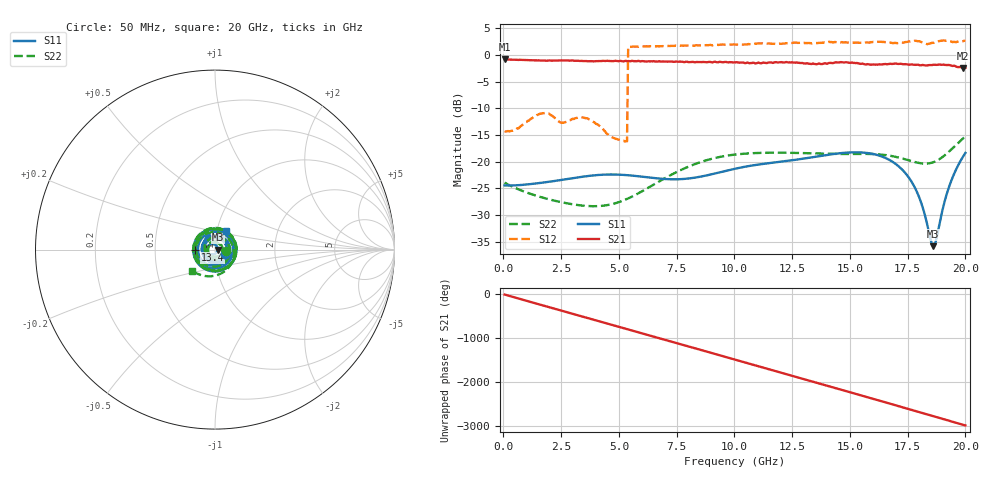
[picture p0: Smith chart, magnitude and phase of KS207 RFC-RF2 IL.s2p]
!Agilent	"Technologies,E8364B,MY43040668,A.07.50.67"
!Agilent	E8364B:	A.07.50.67
!Date:	"Friday,"	June	"03,"	2022	13:37:45
!Correction:	S11(Full	2	"Port(1,2))"
!S21(Full	2	"Port(1,2))"
!S12(Full	2	"Port(1,2))"
!S22(Full	2	"Port(1,2))"
!S2P	File:	Measurements:	"S11,"	"S21,"	"S12,"	S22:
#	Hz	S	dB	R	50
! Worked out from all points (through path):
!   400 points, 50 MHz to 20 GHz, reference 50 ohm
!   highest |S21| = -0.81 dB at 50 MHz (marker M1); lowest = -2.5 dB at 19.9 GHz (marker M2)
!   group delay of S21, straight-line fit = 414 ps
!   lowest |S11| = -35.8 dB at 18.6 GHz (marker M3), VSWR 1.03, Z = 51.6 - j0.0189 ohm
!   |S11| at or under -10 dB: start of sweep to end of sweep
!   |S22| runs from -28.4 to -15.2 dB; largest |S21 - S12| = 0.72
!   S11 on the Smith chart (normalised r, x): 50 MHz: 1.12, -0.05; 13.4 GHz: 0.80, -0.00; 20 GHz: 1.10, +0.23
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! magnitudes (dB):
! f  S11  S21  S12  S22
! 50 MHz  -24.5  -0.8  -14.3  -23.9
! 1.6 GHz  -24.0  -1.1  -11.0  -26.6
! 2.5 GHz  -23.4  -1.0  -12.7  -27.6
! 3.4 GHz  -22.8  -1.1  -11.7  -28.2
! 4.65 GHz  -22.4  -1.2  -15.3  -28.0
! 5.35 GHz  -22.5  -1.2  -16.2  -27.0
! 5.4 GHz  -22.6  -1.2  1.5  -26.9
! 6.7 GHz  -23.2  -1.2  1.6  -23.8
! 8.4 GHz  -22.9  -1.3  1.8  -20.3
! 10.05 GHz  -21.3  -1.4  1.9  -18.7
! 13.35 GHz  -19.2  -1.7  2.2  -18.5
! 13.4 GHz  -19.2  -1.6  2.2  -18.5
! 15.4 GHz  -18.3  -1.6  2.3  -18.6
! 16.7 GHz  -19.7  -1.7  2.3  -18.9
! 17.3 GHz  -21.7  -1.8  2.3  -19.5
! 17.8 GHz  -24.8  -1.9  2.6  -20.1
! 18.15 GHz  -28.6  -1.9  2.3  -20.4
! 18.6 GHz  -35.8  -1.9  2.3  -20.1
! 18.7 GHz  -35.3  -1.9  2.5  -20.0
! 19.25 GHz  -25.3  -1.9  2.6  -18.3
! 19.9 GHz  -19.0  -2.5  2.6  -15.6
! 20 GHz  -18.4  -2.4  2.6  -15.2
